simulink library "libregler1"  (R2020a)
settings: Solver=ode45  StartTime=0.0  StopTime=10.0  RelTol=1e-3

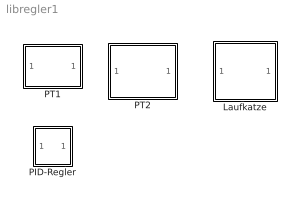
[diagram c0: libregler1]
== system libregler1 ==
  Laufkatze : Subsystem  mask(Laufkatze){mk=100, ml=10, l=1}
      mask prompts: mk "Laufkatzenmasse"; ml "Lastmasse"; l "Seillaenge"
      mask help: Modell einer Laufkatze als Regelstrecke
  PID-Regler : Subsystem  mask(PID-Regler){Kp=10, Ki=20, Kd=5}
      mask prompts: Kp "Proportional"; Ki "Integral"; Kd "Differentiell"
      mask help: Regler mit Proportional-, Integral- und Ableitungsanteil.
  PT1 : Subsystem  mask(PT1){T=2, Kp=5}
      mask prompts: T "Verzoegerungszeit"; Kp "Verstaerkung"
      mask help: Regelstrecke: einfaches Verzoegerungsglied vom PT1-Typ
  PT2 : Subsystem  mask(PT2){D=0.2, om0=1.0, b0=1.0}
      mask prompts: D "Daempfungsgrad"; om0 "Eigenfrequenz"; b0 "Staerke"
      mask help: schwingfaehige Regelstrecke mit Daempfung D Eigenfrequenz om0 Starke b0

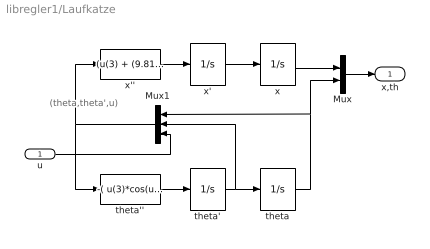
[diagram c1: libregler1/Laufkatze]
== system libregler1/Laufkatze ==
  note: (theta,theta',u)
  u : Inport
  Mux : Mux  Inputs=2
  Mux1 : Mux  Inputs=3
  theta : Integrator
  theta' : Integrator
  theta'' : Fcn  Expr=-( u(3)*cos(u(1)) + (9.81+ l*u(2)^2*cos(u(1)))*ml*sin(u(1)) + 9.81*mk*sin(u(1)) ) / ( (mk + ml*sin(u(1))^2)*l )
  x : Integrator
  x' : Integrator
  x'' : Fcn  Expr=(u(3) + (9.81*cos(u(1)) + l*u(2)^2)*ml*sin(u(1)))/(mk + ml*sin(u(1))^2)
  x,th : Outport
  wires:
  Mux/1 -> x,th/1
  x/1 -> Mux/1
  theta/1 -> Mux/2, Mux1/1
  Mux1/1 -> x''/1, theta''/1
  x'/1 -> x/1
  theta'/1 -> theta/1, Mux1/2
  u/1 -> Mux1/3
  x''/1 -> x'/1
  theta''/1 -> theta'/1

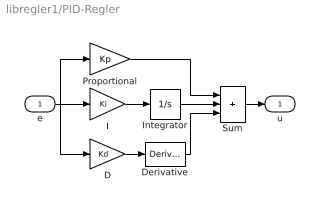
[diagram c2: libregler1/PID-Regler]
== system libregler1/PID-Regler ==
  e : Inport
  D : Gain  Gain=Kd  SaturateOnIntegerOverflow=on
  Derivative : Derivative
  I : Gain  Gain=Ki  SaturateOnIntegerOverflow=on
  Integrator : Integrator
  Proportional : Gain  Gain=Kp  SaturateOnIntegerOverflow=on
  Sum : Sum  Inputs=+++  InputSameDT=on  SaturateOnIntegerOverflow=on
  u : Outport  InitialOutput=0
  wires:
  D/1 -> Derivative/1
  Sum/1 -> u/1
  e/1 -> D/1, Proportional/1, I/1
  Derivative/1 -> Sum/3
  Integrator/1 -> Sum/2
  Proportional/1 -> Sum/1
  I/1 -> Integrator/1

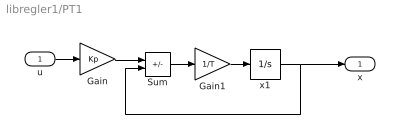
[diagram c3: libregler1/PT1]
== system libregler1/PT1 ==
  u : Inport
  Gain : Gain  Gain=Kp  SaturateOnIntegerOverflow=on
  Gain1 : Gain  Gain=1/T  SaturateOnIntegerOverflow=on
  Sum : Sum  Inputs=+-  SaturateOnIntegerOverflow=on
  x1 : Integrator
  x : Outport
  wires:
  u/1 -> Gain/1
  Gain/1 -> Sum/1
  x1/1 -> x/1, Sum/2
  Sum/1 -> Gain1/1
  Gain1/1 -> x1/1

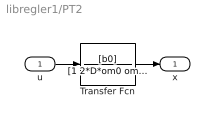
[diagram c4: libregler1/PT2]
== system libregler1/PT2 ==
  u : Inport
  Transfer Fcn : TransferFcn  Numerator=[b0]  Denominator=[1 2*D*om0 om0*om0]
  x : Outport
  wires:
  u/1 -> Transfer Fcn/1
  Transfer Fcn/1 -> x/1
